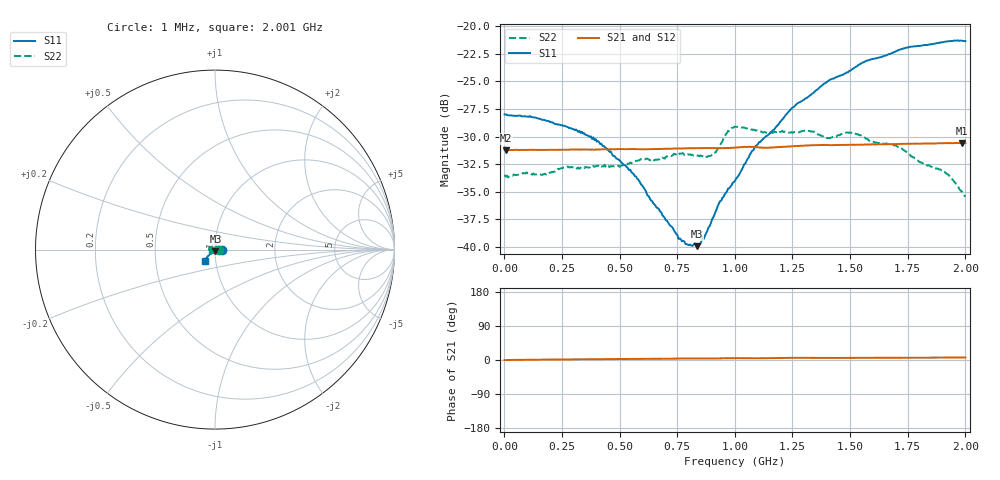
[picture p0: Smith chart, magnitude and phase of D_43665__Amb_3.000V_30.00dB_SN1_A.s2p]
! device id: 43665_
! dir: \\malibu\benchdata\1_engineers\tn_data\43665_75ohm\new\sparar\43665_\amb\3p000v\30p00db
! Serial: 1
! Insertion: A
! Temp: Amb
! VDD: 3.000V
! Attenuation Step: 30.00dB
! IDD: 1.451051e+00mA
! FILE NAME
! DATE 03-27-2009 08:41:02
! CORRECTED  DATA
#  Hz  S  RI  R  75
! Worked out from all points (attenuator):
!   401 points, 1 MHz to 2.001 GHz, reference 75 ohm
!   highest |S21| = -30.58 dB at 1.986 GHz (marker M1); lowest = -31.2 dB at 6 MHz (marker M2)
!   lowest |S11| = -39.9 dB at 836 MHz (marker M3), VSWR 1.02, Z = 75.3 - j1.48 ohm
!   |S11| at or under -10 dB: start of sweep to end of sweep
!   |S22| runs from -35.4 to -29.1 dB; largest |S21 - S12| = 0.00015
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1000000  0.0398 -0.000298  0.0276 5.77e-07  0.0276 7.01e-05  0.0212 -0.000456
6000000  0.0398 -0.000243  0.0274 -0.000102  0.0276 -0.000185  0.0208 0.000115
1.41e8  0.0383 8.52e-05  0.0275 0.000396  0.0275 0.000389  0.0193 0.00905
3.36e8  0.0332 -0.000956  0.0276 0.000847  0.0276 0.0009  0.0124 0.0194
4.16e8  0.0292 -0.00107  0.0276 0.0011  0.0276 0.00108  0.00857 0.0217
5.36e8  0.0226 -0.00286  0.0277 0.0013  0.0277 0.00131  0.00171 0.0238
6.71e8  0.0137 -0.00577  0.0277 0.00171  0.0277 0.00167  -0.00687 0.0239
7.66e8  0.00722 -0.00807  0.0279 0.00183  0.0279 0.00185  -0.0129 0.0231
8.36e8  0.00221 -0.00985  0.028 0.00198  0.028 0.00196  -0.017 0.0196
8.61e8  4.57e-05 -0.0111  0.0279 0.00199  0.028 0.002  -0.0183 0.0182
9.06e8  -0.00411 -0.0129  0.028 0.00205  0.028 0.00204  -0.0216 0.0149
9.71e8  -0.00899 -0.016  0.028 0.00224  0.028 0.00229  -0.03 0.015
1.001e9  -0.0113 -0.0164  0.0281 0.00237  0.0281 0.00239  -0.031 0.0164
1.096e9  -0.0199 -0.0209  0.0282 0.00216  0.0282 0.00221  -0.0311 0.013
1.246e9  -0.031 -0.0288  0.0284 0.00282  0.0285 0.00283  -0.0326 0.00585
1.336e9  -0.0364 -0.0335  0.0287 0.00283  0.0288 0.00283  -0.0333 0.00209
1.406e9  -0.0411 -0.0388  0.0288 0.00268  0.0289 0.00269  -0.0311 -0.00161
1.511e9  -0.0463 -0.0439  0.0289 0.00281  0.0289 0.00284  -0.0324 -0.00471
1.671e9  -0.0523 -0.0532  0.029 0.00302  0.0291 0.00296  -0.0284 -0.00669
1.911e9  -0.0561 -0.0636  0.0293 0.00324  0.0293 0.00324  -0.0209 -0.00655
1.986e9  -0.0555 -0.0654  0.0294 0.00337  0.0294 0.00325  -0.0169 -0.00544
2.001e9  -0.0551 -0.0652  0.0293 0.00341  0.0294 0.00328  -0.0162 -0.00486
